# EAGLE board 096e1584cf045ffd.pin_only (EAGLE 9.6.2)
REV: B

Size 17.78 x 25.4 mm. Coordinates in mm from the lower left corner, seen from the top.
Outline: 0,25.4 0,0 17.78,0 17.78,25.4 12.95,25.4 12.57,25.02 5.46,25.02 5.08,25.4 0,25.4
Copper layers (1*16): Top 0.035mm / dielectric 1.5mm / Bottom 0.035mm
Design rules "adafruit 8-8": minimum track width 6mil, minimum drill 15.5mil, track to track 8mil, track to pad 8mil, pad to pad 8mil, via to via 8mil, smd to smd 8mil, copper to edge 10mil, drill to drill 8mil, minimum pad ring 10mil, minimum via ring 8mil, stop-mask expansion 2mil, vias tented up to drill 20mil, thermal gap 10mil

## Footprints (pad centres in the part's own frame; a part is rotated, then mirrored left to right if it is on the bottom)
0805-NO = smd 1.24 x 1.5: 1 -0.95,0; 2 0.95,0
0603-NO = smd 1.075 x 1: 1 -0.85,0; 2 0.85,0
SHOU_MICROXNJ073 = smd 1 x 1.5: BASE@1 -0.889,-1.721; BASE@2 0.889,-1.721 | smd 0.4 x 1.35: D+ 0,1.86; D- -0.65,1.86; GND 1.3,1.86; ID 0.65,1.86; VBUS -1.3,1.86 | drill 0.8 pad 1.143 offset: SPRT@1 -2.425,1.41; SPRT@2 2.45,1.41 | drill 0.9 pad 2.413 square: SPRT@3 -3.6,-1.265; SPRT@4 3.625,-1.265
1X06-CLEANBIG = drill 1.016 pad 1.778 octagon: 1 -6.35,0; 2 -3.81,0; 3 -1.27,0; 4 1.27,0; 5 3.81,0; 6 6.35,0
SSOP28 = smd 0.4 x 1.5: 1 -4.225,-3.625; 2 -3.575,-3.625; 3 -2.925,-3.625; 4 -2.275,-3.625; 5 -1.625,-3.625; 6 -0.975,-3.625; 7 -0.325,-3.625; 8 0.325,-3.625; 9 0.975,-3.625; 10 1.625,-3.625; 11 2.275,-3.625; 12 2.925,-3.625; 13 3.575,-3.625; 14 4.225,-3.625; 15 4.225,3.625; 16 3.575,3.625; 17 2.925,3.625; 18 2.275,3.625; 19 1.625,3.625; 20 0.975,3.625; 21 0.325,3.625; 22 -0.325,3.625; 23 -0.975,3.625; 24 -1.625,3.625; 25 -2.275,3.625; 26 -2.925,3.625; 27 -3.575,3.625; 28 -4.225,3.625
CHIPLED_0603_NOOUTLINE = smd 0.8 x 0.8: A 0,-0.75; C 0,0.75
SOLDERJUMPER_CLOSEDWIRE = smd 1.168 x 1.6: 1 -0.762,0; 2 0.762,0 | smd 0.635 x 0.203: WIRE 0,0
SOLDERJUMPER_ARROW_NOPASTE = smd 0.762 x 1.524: 1 -1.016,0; 2 1.016,0
FIDUCIAL_1MM = smd 1 x 1: 1 0,0

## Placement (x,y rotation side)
C1  10uF  [0805-NO]  2.92,11.58 270 top
C2  0.1uF  [0603-NO]  2.77,15.37 90 top
C3  0.1uF  [0603-NO]  2.95,18.92 90 top
CN1  MicroB  [SHOU_MICROXNJ073]  8.99,21.97 180 top
FTDI  1x6F  [1X06-CLEANBIG]  8.86,2.41 0 top
IC1  FT232RL  [SSOP28]  9.12,13.34 90 top
PLABEL0  [PLABEL0]  10.57,4.7 90 top
PLABEL1  [PLABEL1]  13.11,4.57 90 top
PLABEL2  [PLABEL2]  8.03,4.83 90 top
PLABEL3  [PLABEL3]  15.77,4.57 90 top
PLABEL4  [PLABEL4]  5.61,4.83 90 top
PLABEL5  [PLABEL5]  3.07,3.56 90 top
PLABEL6  [PLABEL6]  1.27,1.4 90 top
PLABEL7  [PLABEL7]  17.53,1.27 90 top
PLABEL8  [PLABEL8]  1.52,7.24 90 top
PLABEL9  [PLABEL9]  17.42,12.57 90 top
PLABEL10  [PLABEL10]  17.42,15.37 90 top
PLABEL11  [PLABEL11]  8.76,19.3 0 bottom
PLABEL12  [PLABEL12]  8.51,15.75 0 bottom
PLABEL13  [PLABEL13]  8.76,9.65 0 bottom
PLABEL14  [PLABEL14]  14.73,13.72 0 bottom
PLABEL15  [PLABEL15]  14.86,17.53 0 bottom
PLABEL16  [PLABEL16]  2.92,13.59 0 bottom
PLABEL17  [PLABEL17]  2.92,17.65 0 bottom
PLABEL18  [PLABEL18]  2.79,11.3 0 bottom
PLABEL19  [PLABEL19]  14.86,11.43 0 bottom
PLABEL20  [PLABEL20]  8.76,13.84 0 bottom
PLABEL21  [PLABEL21]  8.76,17.65 0 bottom
PLABEL22  [PLABEL22]  8.76,11.43 0 bottom
PLABEL23  [PLABEL23]  9.27,7.11 0 bottom
PLABEL24  [PLABEL24]  8.89,4.95 0 bottom
R1  22  [0603-NO]  13.18,7.24 180 top
R2  10K  [0603-NO]  15.72,19.56 270 top
R3  10K  [0603-NO]  15.72,10.41 90 top
R5  22  [0603-NO]  9.63,7.24 0 top
RX  Green  [CHIPLED_0603_NOOUTLINE]  15.72,16.38 180 top
SJ1  [SOLDERJUMPER_CLOSEDWIRE]  11.66,17.53 0 bottom
SJ2  [SOLDERJUMPER_ARROW_NOPASTE]  11.66,13.72 0 bottom
SJ3  [SOLDERJUMPER_CLOSEDWIRE]  5.94,11.3 180 bottom
SJ4  [SOLDERJUMPER_ARROW_NOPASTE]  6.07,17.53 0 bottom
SJ5  [SOLDERJUMPER_CLOSEDWIRE]  5.94,13.59 0 bottom
SJ6  [SOLDERJUMPER_ARROW_NOPASTE]  11.66,11.43 180 bottom
TX  Red  [CHIPLED_0603_NOOUTLINE]  15.72,13.46 0 top
U$1  FIDUCIAL  [FIDUCIAL_1MM]  16.38,24 270 top
U$2  FIDUCIAL  [FIDUCIAL_1MM]  2.79,8.13 270 top
U$3  [PCBFEAT-REV-040]  2.41,5.84 0 bottom
U$4  [ADAFRUIT_2.5MM]  4.19,23.24 180 top

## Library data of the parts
C1-C3 R1-R3 R5 SJ1 SJ3 SJ5 U$3 U$4 = microbuilder
CN1 = adafruit_electromech; LCSC: C404969
FTDI = adafruit; FORCETHM: 1
IC1 = ftdichip; MPN: FT232RL; OC_FARNELL: 1146032; OC_NEWARK: 91K9918
PLABEL0 PLABEL1-PLABEL24 = pinguin
RX TX = microbuilder; ROT: 270
SJ2 SJ4 SJ6 = microbuilder; BOM: EXCLUDE
U$1 U$2 = adafruit

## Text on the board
Pinguin_tBackup: RX | TX | FTDI Friend! by Adafruit | CTS | VCC | TX | RX | RTS | GND | BLACK | GREEN
Pinguin_bBackup: VCC out | +3V | OR | +5V | Signal logic level | +3V | OR | +5V | RTS | OR | DTR | Pin 6 signal | FTDI Friend | from adafruit!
